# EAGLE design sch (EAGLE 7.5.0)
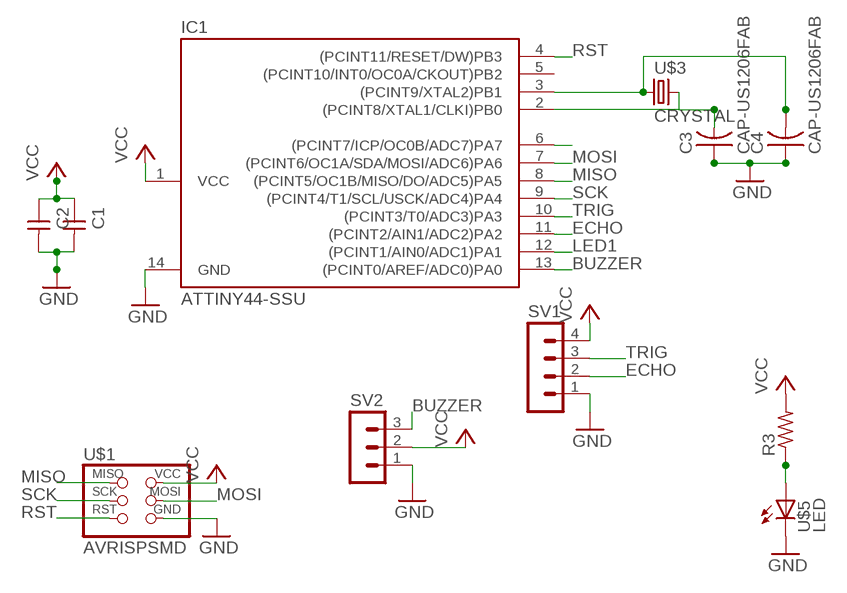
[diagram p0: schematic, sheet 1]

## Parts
C1  CAP-UNPOLARIZEDFAB  [C1206FAB]
C2  CAP-UNPOLARIZEDFAB  [C1206FAB]
C3  CAP-US1206FAB  [C1206FAB]
C4  CAP-US1206FAB  [C1206FAB]
IC1  ATTINY44-SSU  [SOIC14]
R3  RES-US1206FAB  [R1206FAB]
SV1  MA04-1  [MA04-1]
SV2  MA03-1  [MA03-1]
U$1  AVRISPSMD  [2X03SMD]
U$3  CRYSTAL  [2-SMD-5X3MM]
U$5  LED  [LED1206]

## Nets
BUZZER: IC1.13((PCINT0/AREF/ADC0)PA0) SV2.3
ECHO: IC1.11((PCINT2/AIN1/ADC2)PA2) SV1.2
K1: IC1.6((PCINT7/ICP/OC0B/ADC7)PA7) R3.1 U$5.1(A)
LED1: IC1.12((PCINT1/AIN0/ADC1)PA1)
MISO: IC1.8((PCINT5/OC1B/MISO/DO/ADC5)PA5) U$1.1(MISO)
MOSI: IC1.7((PCINT6/OC1A/SDA/MOSI/ADC6)PA6) U$1.4(MOSI)
N$3: C4.2 IC1.3((PCINT9/XTAL2)PB1) U$3.P$1
N$4: C1.2 C2.2 C3.1 C4.1 IC1.14(GND) SV1.1 SV2.1 U$1.6(GND) U$5.2(C) ; supply symbol labelled GND
N$5: C3.2 IC1.2((PCINT8/XTAL1/CLKI)PB0) U$3.P$2
RST: IC1.4((PCINT11/RESET/DW)PB3) U$1.5(RST)
SCK: IC1.9((PCINT4/T1/SCL/USCK/ADC4)PA4) U$1.3(SCK)
TRIG: IC1.10((PCINT3/T0/ADC3)PA3) SV1.3
VCC: C1.1 C2.1 IC1.1(VCC) R3.2 SV1.4 SV2.2 U$1.2(VCC)
Unconnected: IC1.5((PCINT10/INT0/OC0A/CKOUT)PB2)

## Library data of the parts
C1 C2 = fab:CAP-UNPOLARIZED
C3 C4 = fab:CAP-US
IC1 = fab:ATTINY44
R3 = fab:RES-US: Resistor (US Symbol)
SV1 = con-lstb:MA04-1: PIN HEADER; OC_FARNELL: unknown; OC_NEWARK: unknown
SV2 = con-lstb:MA03-1: PIN HEADER; OC_FARNELL: unknown; OC_NEWARK: unknown
U$1 = fab:AVRISP
U$3 = fab:CRYSTAL
U$5 = fab:LED: LED

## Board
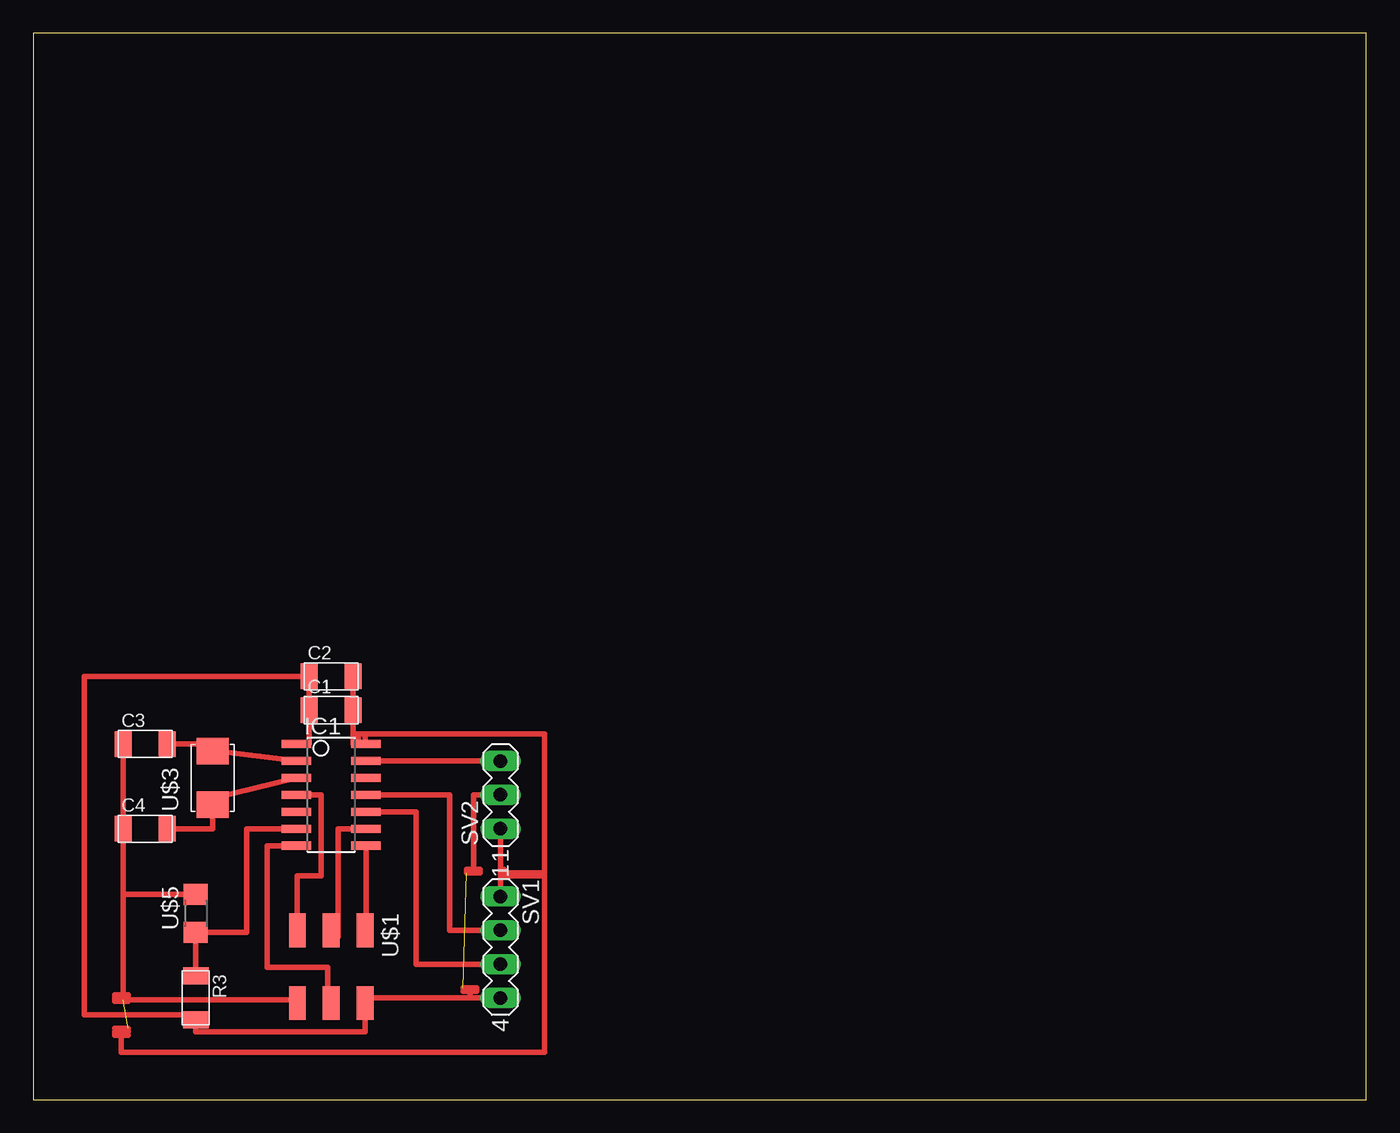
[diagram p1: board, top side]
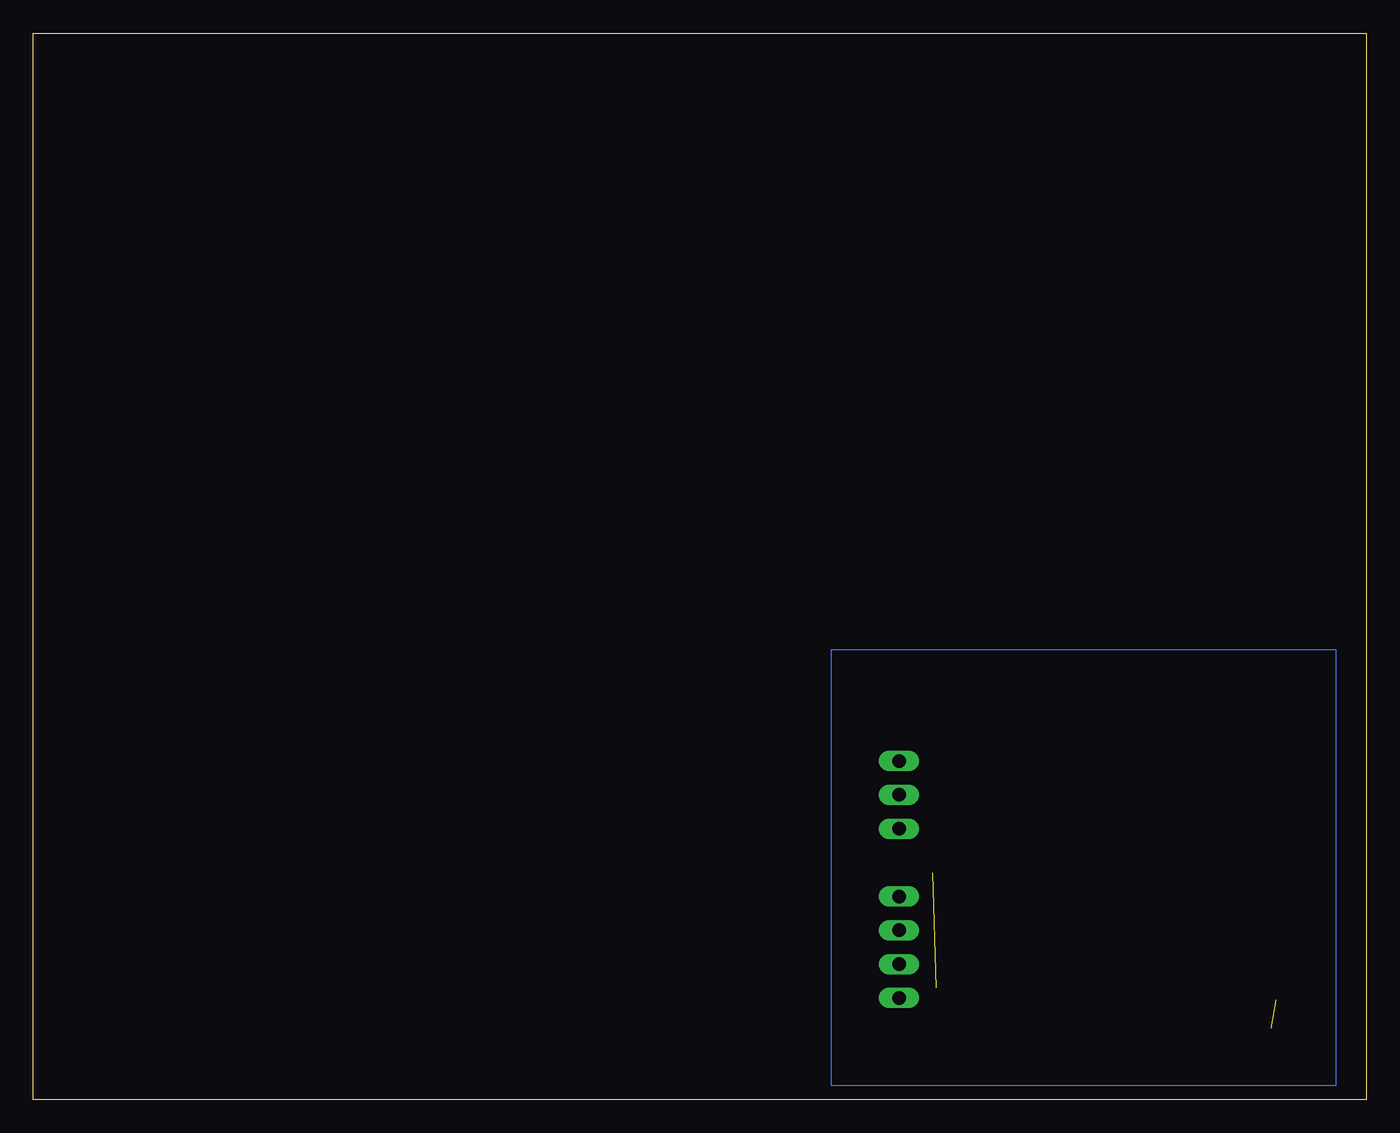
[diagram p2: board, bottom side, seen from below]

Size 100 x 80 mm. Coordinates in mm from the lower left corner, seen from the top.
Outline: 0,0 100,0 100,80 0,80 0,0
Copper layers (1*16): Top 0.035mm / dielectric 1.5mm / Bottom 0.035mm
Design rules "default": minimum track width 10mil, minimum drill 24mil, track to track 8mil, track to pad 8mil, pad to pad 8mil, via to via 8mil, smd to smd 8mil, copper to edge 40mil, drill to drill 8mil, minimum pad ring 10mil, minimum via ring 8mil, stop-mask expansion 4mil, vias tented up to drill 0mil, thermal gap 10mil

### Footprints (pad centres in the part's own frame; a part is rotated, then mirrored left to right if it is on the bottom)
C1206FAB = smd 1.27 x 1.905: 1 -1.651,0; 2 1.651,0
SOIC14 = smd 0.61 x 2.21: 1 -3.81,-2.603; 2 -2.54,-2.603; 3 -1.27,-2.603; 4 0,-2.603; 5 1.27,-2.603; 6 2.54,-2.603; 7 3.81,-2.603; 8 3.81,2.603; 9 2.54,2.603; 10 1.27,2.603; 11 0,2.603; 12 -1.27,2.603; 13 -2.54,2.603; 14 -3.81,2.603
R1206FAB = smd 1.27 x 1.905: 1 -1.651,0; 2 1.651,0
MA04-1 = drill 1.016 long: 1 -3.81,0; 2 -1.27,0; 3 1.27,0; 4 3.81,0
MA03-1 = drill 1.016 long: 1 -2.54,0; 2 0,0; 3 2.54,0
2X03SMD = smd 2.54 x 1.27: 1 -2.54,2.54; 2 2.92,2.54; 3 -2.54,0; 4 2.92,0; 5 -2.54,-2.54; 6 2.92,-2.54
2-SMD-5X3MM = smd 2 x 2.4: P$1 -2,0; P$2 2,0
LED1206 = smd 1.6 x 1.803: 1 -1.422,0; 2 1.422,0

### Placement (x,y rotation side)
C1  22.35,29.21 0 top
C2  22.35,31.75 0 top
C3  8.38,26.67 0 top
C4  8.38,20.32 0 top
IC1  22.35,22.86 270 top
R3  12.19,7.62 270 top
SV1  35.05,11.43 270 top
SV2  35.05,22.86 90 top
U$1  22.35,10.16 270 top
U$3  13.46,24.13 90 top
U$5  12.19,13.97 90 top

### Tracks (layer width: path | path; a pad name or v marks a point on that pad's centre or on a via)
BUZZER
  Top 0.406: SV2.3 IC1.13
ECHO
  Top 0.406: IC1.11 31.24,22.86 31.24,12.7 SV1.2
K1
  Top 0.406: R3.1 U$5.1 16,12.55 16,20.32 IC1.6
MISO
  Top 0.406: U$1.1 24.96,12.7 IC1.8
MOSI
  Top 0.406: U$1.4 22.1,7.24 22.1,9.91 17.53,9.91 17.53,19.05 IC1.7
N$2
  Top 0.406: 6.6,7.62 6.1,7.62 6.1,7.37 7.11,7.37 7.11,7.87 6.1,7.87
N$3
  Top 0.406: IC1.3 13.46,22.61 U$3.P$1 13.46,20.32 C4.2
N$4  (1 unrouted)
  Top 0.406: 6.1,5.33 7.11,5.33 7.11,5.08 6.1,5.08 6.1,4.83 6.6,4.83 | 7.11,4.83 6.6,4.83 | 6.6,4.83 6.6,3.56 38.35,3.56 38.35,16.76 35.05,16.76 | 24.38,26.67 24,26.67 C1.2 C2.2 | SV2.1 35.05,17.27 | 35.05,16.76 SV1.1 | 6.73,15.39 6.73,7.49 19.81,7.49 U$1.6 | 6.73,15.39 C4.1 C3.1 | U$5.2 6.73,15.39 | 35.05,16.76 35.05,17.27 | 35.05,17.27 35.31,17.27 35.31,17.02 38.35,17.02 38.35,27.43 24.89,27.43 | 24.89,27.43 24.13,27.43 24.13,27.18 | 24.89,26.67 24.38,26.67 | 24.38,26.67 24.38,27.18 | IC1.14 24.89,26.67 | 24.89,26.67 24.89,27.43
N$5
  Top 0.406: IC1.2 13.72,26.16 U$3.P$2 13.46,26.67 C3.2
N$6
  Bottom 0.025: 2.29,33.02 2.29,32.51 2.29,1.02 40.13,1.02 40.13,33.78 2.29,33.78 2.29,33.02
RST
  Top 0.406: U$1.5 19.81,16.76 21.59,16.76 21.59,22.86 IC1.4
SCK
  Top 0.406: IC1.9 22.86,20.32 22.86,12.19 22.35,12.19 U$1.3
TRIG
  Top 0.406: IC1.10 28.7,21.59 28.7,10.16 SV1.3
VCC  (1 unrouted)
  Top 0.406: IC1.1 20.7,26.67 C1.1 C2.1 | C2.1 21.08,31.75 | C2.1 3.81,31.75 3.81,6.35 12.19,6.35 R3.2 12.19,5.08 24.89,5.08 U$1.2 24.89,7.62 32.77,7.62 | SV1.4 32.77,7.62 | SV2.2 33.02,22.86 33.02,17.27 | 33.02,17.27 33.53,17.27 33.53,17.02 32.51,17.02 32.51,17.27 33.02,17.27 | 32.77,7.62 32.77,8.13 | 32.77,8.13 32.26,8.13 | 32.77,8.13 33.27,8.13 33.27,8.38 32.26,8.38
